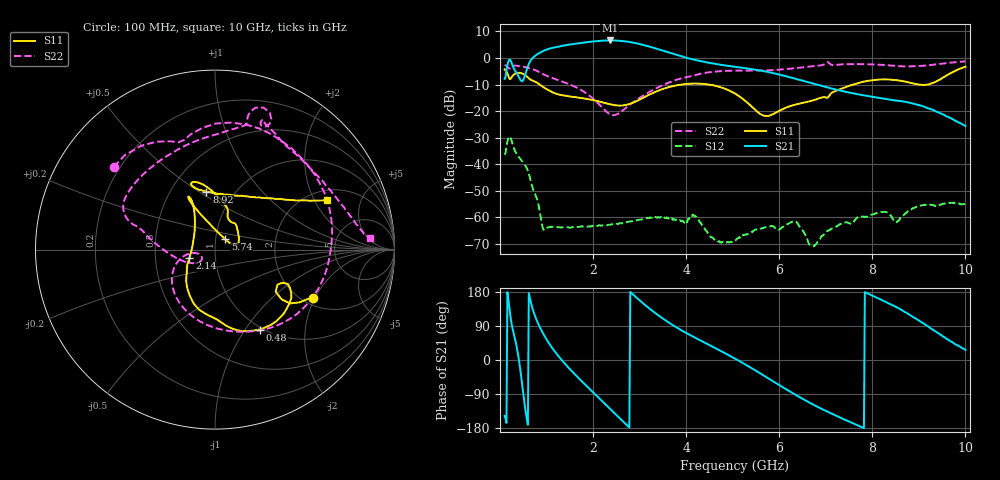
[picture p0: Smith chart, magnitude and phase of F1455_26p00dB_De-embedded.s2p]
! Integrated Device Technology
! Corporate Headquarters
! 6024 Silver Creek Valley Road
! San Jose, CA 95138  USA
! Phone:  1-408-284-8200
! Toll Free:  1-800-223-1366
! Webpage:  http://www.idt.com/
! Timing and RF Division
! 515 Groton Road, Suite 102
! Westford, MA 01886-6024
! Device:  F1455
! Description: 6-bit 0.5 dB Transmit Variable Gain Amplifier
! Frequency:  1400.0 -  2300.00 MHz
! Package:  6x6 mm Thin QFN Plastic Package: 28 pin
! State:  52
! Atten State:  26.0 dB
! Voltage:  +5.00 Volts
! Current:  217.630 mA
! Data:  The device was measured on a the F1455 evaluation board which has
!  individual transmission lines to the RF pins.  Data was collected
!  using a calibrated network analyzer.  The evaluation board was
!  de-embedded using a TRL calibration technique.
!  The reference plane is the edge of the package pin.
!  Pin  1 = CSb
!  Pin  2 = DATA
!  Pin  3 = CLK
!  Pin  4 = RSET
!  Pin  5 = GND
!  Pin  6 = RFIN  = Port 1
!  Pin  7 = GND
!  Pin  8 = NC
!  Pin  9 = NC
!  Pin 10 = NC
!  Pin 11 = NC
!  Pin 12 = NC
!  Pin 13 = NC
!  Pin 14 = /STBY
!  Pin 15 = GND
!  Pin 16 = RFOUT  = Port 2
!  Pin 17 = GND
!  Pin 18 = NC
!  Pin 19 = NC
!  Pin 20 = NC
!  Pin 21 = GND
!  Pin 22 = NC
!  Pin 23 = GND
!  Pin 24 = NC
!  Pin 25 = NC
!  Pin 26 = NC
!  Pin 27 = GND
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# GHz S dB R 50
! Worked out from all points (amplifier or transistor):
!   496 points, 100 MHz to 10 GHz, reference 50 ohm
!   highest |S21| = 6.6 dB at 2.36 GHz (marker M1)
!   |S21| within 3 dB of that: 1.082 GHz to 3.346 GHz (2.263 GHz wide, 102 % of centre)
!   unconditionally stable (mu >= 1): start of sweep to end of sweep
!   at 1.74 GHz: K = 347.91, MAG = 6.1 dB, |S12| = -63.4 dB
!   at 5.06 GHz: K = 1269.15, MAG = -1.4 dB, |S12| = -68.7 dB
!   at 10 GHz: K = 722.58, MAG = -16.9 dB, |S12| = -54.9 dB
!   S11 on the Smith chart (normalised r, x): 100 MHz: 2.27, -1.94; 480 MHz: 0.97, -1.17; 2.14 GHz: 0.75, -0.07; 5.74 GHz: 1.11, +0.13; 8.92 GHz: 0.74, +0.54; 10 GHz: 2.44, +2.55
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0.1  -4.30 -26.1  -7.88 -147.5  -36.40 47.3  -2.75 140.7
0.18  -6.70 -36.8  -1.33 161.1  -30.18 -6.4  -3.70 112.5
0.26  -6.98 -25.2  -2.28 88.9  -31.66 -77.1  -3.33 96.0
0.38  -5.63 -42.6  -6.28 21.4  -36.68 -118.8  -2.98 58.1
0.48  -5.84 -60.7  -8.74 -69.1  -38.93 -150.6  -3.23 31.3
0.66  -8.16 -88.1  -0.93 154.0  -46.22 140.4  -4.02 -11.4
0.8  -9.32 -105.9  1.39 101.7  -53.32 111.4  -4.91 -42.8
0.94  -11.07 -121.8  2.73 67.2  -64.66 120.0  -6.20 -69.1
1.32  -13.98 -141.8  4.52 0.9  -63.74 113.1  -8.76 -120.2
1.76  -15.06 -151.2  5.72 -56.4  -63.30 80.7  -12.22 -156.9
2.14  -16.41 -161.1  6.44 -101.9  -62.90 66.0  -17.64 -171.4
2.36  -17.39 -172.9  6.60 -128.3  -62.77 61.1  -21.14 -160.6
2.78  -17.35 150.0  6.03 -178.1  -61.51 51.9  -17.79 -144.6
3.4  -12.30 118.5  3.31 118.1  -59.86 29.5  -11.05 -179.0
4.08  -9.68 116.1  -0.25 66.2  -59.62 15.7  -6.94 163.4
5.06  -13.49 112.0  -3.34 3.1  -68.69 31.2  -4.75 147.9
5.74  -21.84 45.5  -5.20 -46.5  -63.53 25.5  -4.67 119.8
6.34  -17.55 14.2  -7.77 -91.0  -61.46 -18.1  -3.85 89.4
6.7  -16.09 34.6  -9.50 -115.7  -70.44 -153.8  -3.13 78.4
8.36  -8.09 109.5  -15.67 148.9  -58.57 66.5  -2.78 62.2
8.92  -9.72 98.3  -17.32 109.8  -56.19 86.3  -3.11 39.7
10  -3.30 24.0  -25.63 26.3  -54.95 16.9  -1.28 4.4
